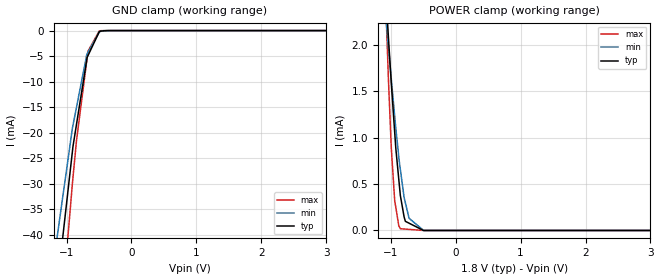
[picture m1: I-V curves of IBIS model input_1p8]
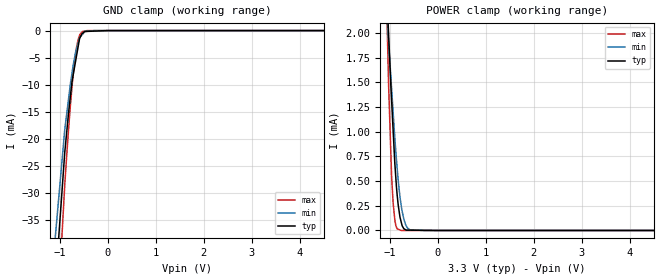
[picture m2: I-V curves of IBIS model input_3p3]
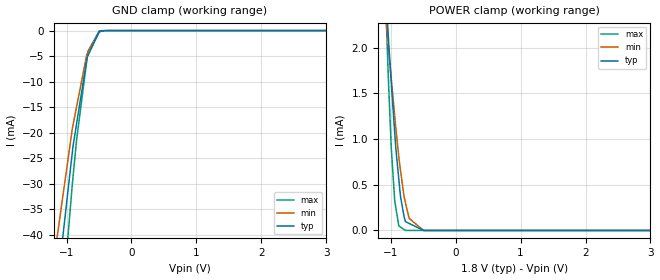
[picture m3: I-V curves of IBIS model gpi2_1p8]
|Texas Instruments Incorporated
| 4-Wire Touch Screen Controller with Low-Power Mono ADC/Stereo DAC
| Marketing part#   Digital Voltage Range   Package-type   #pins
| TSC2117IRGZR   1.1V - 3.6V   VQFN   48
| TSC2117IRGZT   1.1V - 3.6V   VQFN   48
[IBIS Ver]   3.2
[File name]   tsc2117.ibs
|SIMDE Ver   V3.0 - 201101 - RHL4 - Build 457
[File Rev]   1.1
[Date]   9/15/2011
[Source]
| Texas Instruments Incorporated.
| Analog-eLab Design Center, HPA
| 12500 TI Blvd
| Dallas, TX -75243
| e-mail: elab_scm_ibis@list.ti.com
[Notes]   Revision History:
| Rev 1.1: 9/15/2011
| - Updated C_comp values without Bondpad.
| Rev 1.0: 8/24/2011
| - Initial version of the model
| - Model generated from simulations in TISPICE
| - Model matched to SPICE simulation
| - C_comp although listed in numerical order of value are
|   obtained from varying PVT conditions. For PVT conditions for
|   each specific value refer the buffer description under
|   respective [Model]. IBIS model user is responsible for using
|   appropriate C_comp to simulate for Signal Integrity.
| - Model names with a trailing _1p8 contains the model for
|   1.8V [1.62V and 1.98V].Model names with a trailing _3p3
|   contains the model for 3.3V [3.0V and 3.6V].
|*  EXCEPTION:   *
|*  - For model gpi2, there will be a leakage current in the GND   *
|*   clamp I-V Table because of the pullup on pad.   *
|*  - For model scl_3p3 and sda_3p3, there will be a leakage current in *
|*   the POWER clamp I-V Table because of the pulldown on pad.   *
[Disclaimer]
| This model is designed as an aid for customers of Texas Instruments.
| TI and its licensors and suppliers make no warranties, either expressed
| or implied, with respect to this  model, including the warranties of
| merchantability or fitness for a particular purpose. The model is
| provided solely on an "as is" basis. The entire risk as to its quality
| and performance is with the customer.
[Copyright]
 (C) Copyright 2011 Texas Instruments Incorporated.All rights reserved.
|   TSC2117
[Component]   TSC2117
[Manufacturer]   TI
[Package]   |48 VQFN   -  RGZ package
|   typ   min   max
R_pkg   0.13043   0.06420   0.17475
L_pkg   2.11650nH   1.57946nH   2.79981nH
C_pkg   0.23951pF   0.20186pF   0.30126pF
[Pin]  signal_name   model_name   R_pin   L_pin   C_pin
1   MISO   MISO   0.14319   2.24943nH  0.23522pF
2   MOSI   INPUT   0.12501   1.92928nH  0.21836pF
3   _SS   INPUT   0.11730   1.79434nH  0.20902pF
4   SCLK   INPUT   0.11235   1.70804nH  0.20355pF
5   GPIO1   I/O   0.11071   1.67950nH  0.20186pF
6   GPIO2   I/O   0.11256   1.71170nH  0.20432pF
7   IOVSS   GND   0.11774   1.80209nH  0.21256pF
8   IOVDD   POWER   0.06302   1.50017nH  0.28212pF
9   DVDD   POWER   0.06816   1.69777nH  0.29480pF
10   SDOUT   SDOUT   0.14447   2.27104nH  0.24913pF
11   SDIN   INPUT   0.16035   2.55117nH  0.27539pF
12   WCLK   I/O   0.17144   2.74752nH  0.27606pF
13   BCLK   I/O   0.17348   2.78271nH  0.26217pF
14   MCLK   INPUT   0.15799   2.50827nH  0.24793pF
15   SDA   SDA   0.15181   2.39843nH  0.24067pF
16   SCL   SCL   0.14822   2.33443nH  0.23000pF
17   VOL/MICDET   TERM   0.15686   2.48810nH  0.24636pF
18   MICBIAS   TERM   0.14949   2.35719nH  0.24768pF
19   MIC   TERM   0.14637   2.30119nH  0.24477pF
20   AUX1   TERM   0.14704   2.31220nH  0.24553pF
21   AUX2   TERM   0.15133   2.38693nH  0.24529pF
22   AVSS   GND   0.15715   2.48904nH  0.25102pF
23   AVDD   POWER   0.16627   2.64986nH  0.26629pF
24   VBAT   TERM   0.17475   2.79981nH  0.26680pF
25   VREF   TERM   0.16260   2.58410nH  0.25365pF
26   TSVSS   GND   0.14451   2.26427nH  0.24339pF
27   YN   TERM   0.13277   2.05724nH  0.23297pF
28   XN   TERM   0.12062   1.84354nH  0.21871pF
29   DVSS   GND   0.11400   1.72751nH  0.20646pF
30   YP   TERM   0.11101   1.67519nH  0.20574pF
31   XP   TERM   0.11246   1.70039nH  0.20739pF
32   TSVDD   POWER   0.11725   1.78460nH  0.21715pF
33   SPLN   TERM   0.06420   1.57946nH  0.28715pF
34   SLVSS   GND   0.06966   1.76606nH  0.29644pF
35   SLVDD   POWER   0.07325   1.89164nH  0.30852pF
36   SPLP   TERM   0.07643   1.98179nH  0.30126pF
37   SPRN   TERM   0.07087   1.80471nH  0.28107pF
38   SRVDD   POWER   0.06793   1.69889nH  0.28808pF
39   SRVSS   GND   0.06500   1.59821nH  0.26356pF
40   SPRP   TERM   0.06611   1.63862nH  0.25779pF
41   HPL   TERM   0.12931   1.99780nH  0.22385pF
42   HVDD   POWER   0.11949   1.82650nH  0.21846pF
43   HVSS   GND   0.11418   1.73479nH  0.21061pF
44   HPR   TERM   0.11426   1.73760nH  0.20492pF
45   GPI3   INPUT   0.11601   1.76853nH  0.21025pF
46   GPI2   GPI2   0.12396   1.90884nH  0.22266pF
47   GPI1   INPUT   0.13380   2.08237nH  0.23865pF
48   _RESET   INPUT   0.14562   2.29122nH  0.24710pF
49   THERMAL_PAD   NC   0.00005   0.00060nH  1.63026pF
[Pin Mapping]  pulldown_ref pullup_ref gnd_clamp_ref power_clamp_ref
1   GNDBUS1   PWRBUS1
2   GNDBUS4   PWRBUS1
3   GNDBUS4   PWRBUS1
4   GNDBUS4   PWRBUS1
5   GNDBUS1   PWRBUS1
6   GNDBUS1   PWRBUS1
7   GNDBUS1   NC
8   NC   PWRBUS1
9   NC   PWRBUS2
10   GNDBUS1   PWRBUS1
11   GNDBUS4   PWRBUS1
12   GNDBUS1   PWRBUS1
13   GNDBUS1   PWRBUS1
14   GNDBUS4   PWRBUS1
15   GNDBUS1   NC
16   GNDBUS1   NC
17   GNDBUS4   PWRBUS3
18   GNDBUS4   PWRBUS3
19   GNDBUS4   PWRBUS3
20   GNDBUS4   PWRBUS3
21   GNDBUS4   PWRBUS3
22   GNDBUS2   NC
23   NC   PWRBUS3
24   GNDBUS4   NC
25   GNDBUS4   PWRBUS3
26   GNDBUS3   NC
27   GNDBUS4   NC
28   GNDBUS4   NC
29   GNDBUS4   NC
30   GNDBUS4   NC
31   GNDBUS4   NC
32   NC   PWRBUS4
33   GNDBUS4   NC
34   GNDBUS5   NC
35   NC   PWRBUS5
36   GNDBUS4   NC
37   GNDBUS4   NC
38   NC   PWRBUS6
39   GNDBUS6   NC
40   GNDBUS4   NC
41   GNDBUS4   PWRBUS7
42   NC   PWRBUS7
43   GNDBUS7   NC
44   GNDBUS4   PWRBUS7
45   GNDBUS4   PWRBUS1
46   GNDBUS4   PWRBUS1
47   GNDBUS4   PWRBUS1
48   GNDBUS4   PWRBUS1
49   NC   NC
|   Model Selectors
[Model Selector] INPUT
input_1p8  1.8V digital input
input_3p3  3.3V digital input
[Model Selector] GPI2
gpi2_1p8  1.8V digital input
gpi2_3p3  3.3V digital input
[Model Selector] SCL
scl_1p8  1.8V digital input
scl_3p3  3.3V digital input
[Model Selector] MISO
miso_1p8  1.8V digital 3-state
miso_3p3  3.3V digital 3-state
[Model Selector] SDOUT
sdout_1p8  1.8V digital 3-state
sdout_3p3  3.3V digital 3-state
[Model Selector] I/O
io_1p8  1.8V digital I/O
io_3p3  3.3V digital I/O
[Model Selector] SDA
sda_1p8  1.8V digital I/O Open Drain
sda_3p3  3.3V digital I/O Open Drain
[Model Selector] TERM
term_1-8V  1.8V nominal termination
term_3-3V  3.3V nominal termination
[Model] term_1-8V
Model_type Terminator
C_comp   1.0e-20F  1.0e-20F  1.0e-20F
|   typ   min   max
[Voltage Range]   1.8V   1.62V   1.98V
[POWER Clamp Reference]   1.8V   1.62V   1.98V
[GND Clamp Reference]   0V   0V   0V
|Ambient Temperature   25   85   -40
|Junction Temperature
[Temperature Range]   48   108   -40
[Model] term_3-3V
Model_type Terminator
C_comp   1.0e-20F  1.0e-20F  1.0e-20F
|   typ   min   max
[Voltage Range]   3.3V   3.0V   3.6V
[POWER Clamp Reference]   3.3V   3.0V   3.6V
[GND Clamp Reference]   0V   0V   0V
|Ambient Temperature   25   85   -40
|Junction Temperature
[Temperature Range]   48   108   -40
| Models and submodels in the file (16): input_1p8 (Input), input_3p3 (Input), gpi2_1p8 (Input), gpi2_3p3 (Input), scl_1p8 (Input), scl_3p3 (Input), miso_1p8 (3-state), miso_3p3 (3-state), sdout_1p8 (3-state), sdout_3p3 (3-state), io_1p8 (I/O), io_3p3 (I/O), sda_1p8 (I/O_open_drain), sda_3p3 (I/O_open_drain), term_1-8V (Terminator), term_3-3V (Terminator)
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|   input_1p8 Model
[Model]   input_1p8
Model_type   Input
Vinl = 0.54
Vinh = 1.26
|   typ   min   max
|   (nom PVT)   (fast PVT)   (slow PVT)
|C_comp from frequency sweep method (F=25MHz)
|Average
|C_comp   1.556e-12   1.517e-12   1.563e-12
|C_comp from LC tank measurement(L=1nH)
|Average
|Resonant Frequency(Hz)   4.930e+09   4.940e+09   4.920e+09
C_comp   1.043e-12   1.039e-12   1.047e-12
| Where nom  PVT is Nominal Process, 1.8V, 48C
|   Fast PVT is Strong Process,  1.98V, -40C
|   Slow PVT is Weak Process,   1.62V, 108C
[Model Spec]
|Subparameter   typ   min   max
Vinh   1.26   1.134   1.386
Vinl   0.54   0.486   0.594
[Voltage Range]   1.8   1.62   1.98
|Ambient Temperature   25   85   -40
|Junction Temperature
[Temperature Range]   48   108   -40
[Power Clamp Reference]   1.8   1.62   1.98
[GND Clamp Reference]   0   0   0
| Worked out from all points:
|   GND clamp passes 1 mA (typ) near -0.52 V on its own axis
|   POWER clamp passes 1 mA (typ) near -0.93 V on its own axis
[GND Clamp]
|   Voltage   I(typ)   I(min)   I(max)
-1.8V     -219.3mA   -110.6mA   -356.2mA
-1.156V   -51.67mA   -41.55mA   -67.42mA
-910.4mV  -23.84mA   -19.25mA   -30.15mA
-900mV    -22.69mA   -18.55mA   -28.74mA
-845.5mV  -18.32mA   -14.99mA   -21.51mA
-686.9mV  -5.629mA   -4.649mA   -5.784mA
-682.2mV  -5.254mA   -4.542mA   -5.32mA
-669.2mV  -4.905mA   -4.246mA   -4.034mA
-495mV    -214.3uA   -267.7uA   -60.09uA
-307.8mV  -1.174uA   -3.108uA   -82.49nA
3.6V      0A         0A         0A
[POWER Clamp]
|   Voltage   I(typ)   I(min)   I(max)
-1.8V     11.89mA    8.634mA    19.35mA
-1.085V   2.686mA    2.385mA    2.616mA
-1.035V   2.081mA    1.973mA    1.633mA
-990mV    1.577mA    1.628mA    881.4uA
-938.5mV  1.059mA    1.234mA    323.2uA
-919.8mV  874.1uA    1.094mA    242.3uA
-875.2mV  549.7uA    793.1uA    49.36uA
-851.4mV  377uA      658uA      18.85uA
-774mV    98.6uA     299.2uA    14.76uA
-717.7mV  78.69uA    132uA      11.78uA
-494.1mV  14.81nA    598.6nA    0A
3.6V      0A         0A         0A
|   input_3p3 Model
[Model]   input_3p3
Model_type   Input
Vinl = 0.99
Vinh = 2.31
|   typ   min   max
|   (nom PVT)   (fast PVT)   (slow PVT)
|C_comp from frequency sweep method (F=25MHz)
|Average
|C_comp   1.462e-12   1.456e-12   1.467e-12
|C_comp from LC tank measurement(L=1nH)
|Average
|Resonant Frequency(Hz)   5.080e+09   5.110e+09   5.079e+09
C_comp   9.825e-13   9.710e-13   9.829e-13
| Where nom  PVT is Nominal Process, 3.3V, 48C
|   Fast PVT is Strong Process,  3.6V, -40C
|   Slow PVT is Weak Process,   3V, 108C
[Model Spec]
|Subparameter   typ   min   max
Vinh   2.31   2.1   2.52
Vinl   0.99   0.9   1.08
[Voltage Range]   3.3   3   3.6
|Ambient Temperature   25   85   -40
|Junction Temperature
[Temperature Range]   48   108   -40
[Power Clamp Reference]   3.3   3   3.6
[GND Clamp Reference]   0   0   0
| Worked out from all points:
|   GND clamp passes 1 mA (typ) near -0.56 V on its own axis
|   POWER clamp passes 1 mA (typ) near -0.93 V on its own axis
[GND Clamp]
|   Voltage   I(typ)   I(min)   I(max)
-3.3V     -1.744A    -1.584A    -1.955A
-1.498V   -97.24mA   -78.51mA   -125mA
-897.6mV  -22.45mA   -18.25mA   -28.4mA
-788.4mV  -12.73mA   -10.42mA   -14.69mA
-745.8mV  -9.337mA   -7.78mA    -10.25mA
-698.4mV  -6.949mA   -5.254mA   -6.058mA
-622.8mV  -3.141mA   -2.43mA    -1.773mA
-590.7mV  -1.524mA   -1.412mA   -920.3uA
-532.8mV  -547.8uA   -745.5uA   -189uA
-474mV    -165.4uA   -162.8uA   -75.77uA
-285mV    -99uA      -1.687uA   -4.35uA
6.6V      0A         0A         0A
[POWER Clamp]
|   Voltage   I(typ)   I(min)   I(max)
-3.3V     32.07mA    22.39mA    56.05mA
-1.092V   2.754mA    2.444mA    2.811mA
-1.03V    2.019mA    1.931mA    1.532mA
-964.8mV  1.325mA    1.442mA    561.5uA
-932.4mV  1.017mA    1.2mA      280.4uA
-896.4mV  677.8uA    930.6uA    104uA
-858mV    413.8uA    684.7uA    27.87uA
-825mV    253.1uA    501.2uA    12.39uA
-766.8mV  91.1uA     263uA      409.3nA
-675mV    8.087uA    63uA       185nA
-579mV    3.281uA    6.324uA    109.7nA
6.6V      0A         0A         0A
|   gpi2_1p8 Model
[Model]   gpi2_1p8
Model_type   Input
Vinl = 0.54
Vinh = 1.26
|   typ   min   max
|   (nom PVT)   (fast PVT)   (slow PVT)
|C_comp from frequency sweep method (F=25MHz)
|Average
|C_comp   1.654e-12   1.603e-12   1.680e-12
|C_comp from LC tank measurement(L=1nH)
|Average
|Resonant Frequency(Hz)   4.930e+09   4.940e+09   4.920e+09
C_comp   1.043e-12   1.039e-12   1.047e-12
| Where nom  PVT is Nominal Process, 1.8V, 48C
|   Fast PVT is Strong Process,  1.98V, -40C
|   Slow PVT is Weak Process,   1.62V, 108C
[Model Spec]
|Subparameter   typ   min   max
Vinh   1.26   1.134   1.386
Vinl   0.54   0.486   0.594
[Voltage Range]   1.8   1.62   1.98
|Ambient Temperature   25   85   -40
|Junction Temperature
[Temperature Range]   48   108   -40
[Power Clamp Reference]   1.8   1.62   1.98
[GND Clamp Reference]   0   0   0
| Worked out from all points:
|   GND clamp passes 1 mA (typ) near -0.52 V on its own axis
|   POWER clamp passes 1 mA (typ) near -0.93 V on its own axis
[GND Clamp]
|   Voltage   I(typ)   I(min)   I(max)
-1.8V     -219.3mA   -110.6mA   -356.2mA
-1.156V   -51.67mA   -41.55mA   -67.42mA
-910.4mV  -23.84mA   -19.25mA   -30.15mA
-900mV    -22.69mA   -18.55mA   -28.74mA
-845.5mV  -18.32mA   -14.99mA   -21.51mA
-686.9mV  -5.629mA   -4.649mA   -5.784mA
-682.2mV  -5.254mA   -4.542mA   -5.32mA
-669.2mV  -4.905mA   -4.246mA   -4.034mA
-495mV    -214.3uA   -267.7uA   -60.13uA
-307.8mV  -1.203uA   -3.124uA   -139.3nA
3.6V      0A         0A         0A
[POWER Clamp]
|   Voltage   I(typ)   I(min)   I(max)
-1.8V     12mA       8.729mA    19.47mA
-1.085V   2.716mA    2.417mA    2.637mA
-1.035V   2.105mA    2.001mA    1.647mA
-990mV    1.597mA    1.652mA    890.5uA
-938.5mV  1.073mA    1.253mA    327.1uA
-875.2mV  560.7uA    807.2uA    49.98uA
-849.6mV  374uA      660.8uA    37.73uA
-793.8mV  150.1uA    366.1uA    10.98uA
-772.2mV  96.59uA    301.1uA    631.4nA
-716mV    77.03uA    132.2uA    515.8nA
-494.1mV  52.98nA    641.4nA    60.88nA
3.6V      0A         0A         0A
